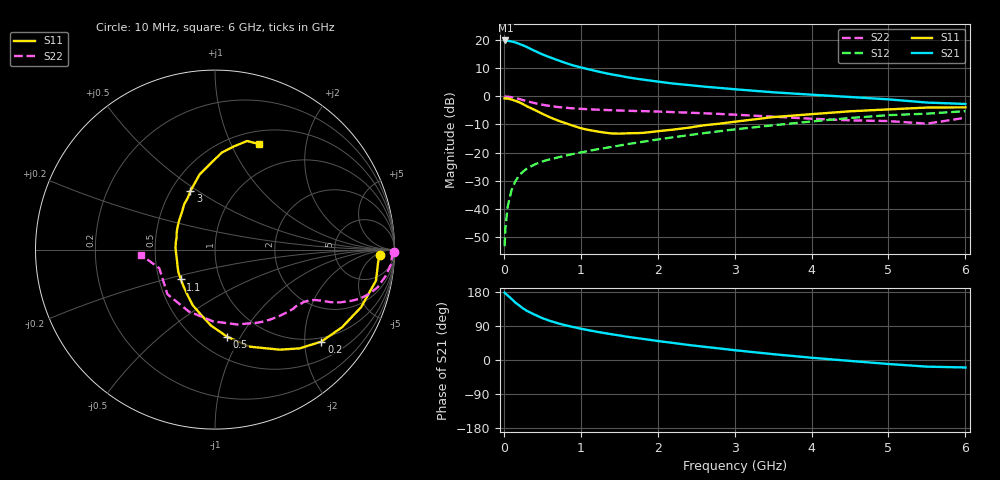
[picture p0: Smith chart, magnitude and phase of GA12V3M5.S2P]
! Infineon Technologies  Discrete & RF Semiconductors
! BF775
! Si NPN RF Bipolar Junction Transistor in SOT23
! VCE = 12 V  IC = 3.5 mA
! Common Emitter S-Parameters:  May  1996
# GHz  S  MA  R  50
!  f  S11  S21  S12  S22
! GHz  MAG  ANG  MAG  ANG  MAG  ANG  MAG  ANG
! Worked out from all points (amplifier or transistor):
!   36 points, 10 MHz to 6 GHz, reference 50 ohm
!   highest |S21| = 19.8 dB at 20 MHz (marker M1)
!   |S21| within 3 dB of that: start of sweep to 349.8 MHz
!   unconditionally stable (mu >= 1): 1.007 GHz to 3.047 GHz
!   at 250 MHz: K = 0.38, MSG = 22.4 dB, |S12| = -26.7 dB
!   at 1.4 GHz: K = 1.10, MAG = 10.9 dB, |S12| = -18.0 dB
!   at 6 GHz: K = 0.88, MSG = 1.3 dB, |S12| = -5.3 dB
!   S11 on the Smith chart (normalised r, x): 10 MHz: 20, -8; 200 MHz: 0.90, -2.39; 500 MHz: 0.69, -0.88; 1.1 GHz: 0.65, -0.23; 3 GHz: 0.63, +0.47; 6 GHz: 0.65, +1.28
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0.01  0.9195 -2.0  9.748 177.8  0.0022 84.5  0.9968 -0.8
0.02  0.9118 -4.1  9.768 175.6  0.0046 87.8  0.987 -1.9
0.05  0.9135 -10.9  9.626 170.3  0.0111 82.1  0.9847 -4.7
0.1  0.8751 -21.5  9.4 161.2  0.0217 78.0  0.9611 -8.9
0.15  0.8297 -31.4  9.004 151.5  0.0312 72.2  0.9307 -13.0
0.2  0.7837 -40.8  8.484 143.9  0.0397 68.3  0.8954 -15.9
0.25  0.725 -49.4  8.008 136.2  0.0463 64.1  0.8556 -18.5
0.3  0.664 -57.1  7.466 129.6  0.0524 61.8  0.8163 -20.4
0.4  0.574 -70.4  6.401 119.8  0.0619 58.0  0.756 -22.9
0.5  0.4906 -82.0  5.529 110.5  0.0699 55.8  0.7092 -24.4
0.6  0.4233 -93.1  4.905 103.2  0.0763 54.7  0.6717 -25.3
0.7  0.3732 -101.7  4.37 97.1  0.0821 54.9  0.6457 -26.0
0.8  0.3344 -111.7  3.905 91.7  0.0887 54.6  0.6252 -26.7
1.1  0.253 -138.9  3.013 78.7  0.1074 55.3  0.5888 -29.1
1.3  0.2277 -156.6  2.606 71.3  0.1202 56.1  0.5724 -30.9
1.6  0.2203 177.4  2.181 61.4  0.1413 56.6  0.5534 -34.3
2.2  0.2564 141.5  1.681 45.0  0.1876 55.9  0.5241 -43.2
3  0.3537 112.8  1.333 25.9  0.2586 51.7  0.4722 -59.5
3.5  0.4273 101.6  1.178 15.4  0.3061 47.2  0.435 -73.5
4.5  0.5418 86.0  0.971 -2.4  0.4121 36.2  0.3742 -113.1
5.5  0.6309 73.5  0.774 -17.5  0.4918 20.4  0.3274 -161.6
6  0.637 67.5  0.731 -19.7  0.5455 16.1  0.4158 -176.2
